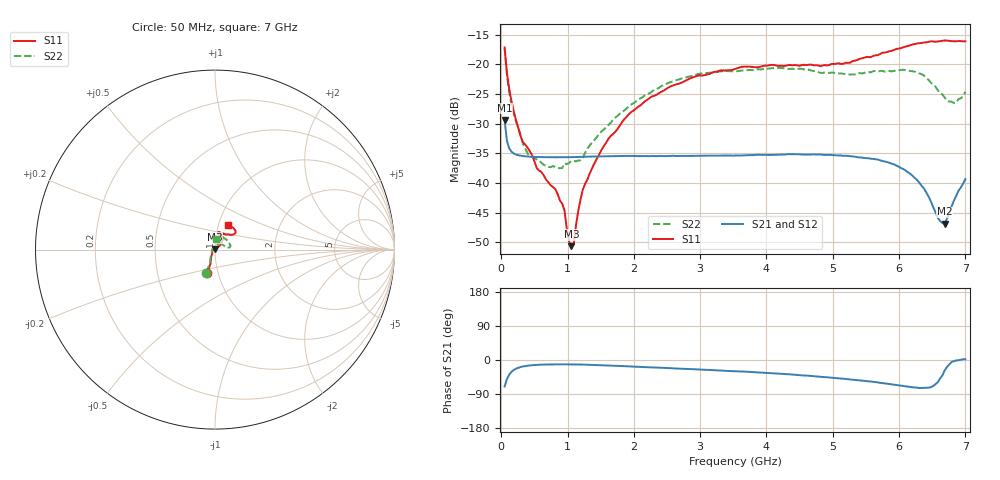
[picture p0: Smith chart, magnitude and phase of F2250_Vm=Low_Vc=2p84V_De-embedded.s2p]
! Integrated Device Technology
! Corporate Headquarters
! 6024 Silver Creek Valley Road
! San Jose, CA 95138  USA
! Phone:  1-408-284-8200
! Toll Free:  1-800-223-1366
! Webpage:  http://www.idt.com/
! Timing and RF Division
! 515 Groton Road, Suite 102
! Westford, MA 01886-6024
! Device:  F2250
! Description: Voltage Variable RF Attenuator
! Frequency:  50.0 -  6000.00 MHz
! Package:  3x3 mm Thin QFN Plastic Package: 16 pin
! Ports:  2 RF, 3 DC
!  Pin  1  = GND
!  Pin  2  = NC
!  Pin  3  = RF1  = Port 1
!  Pin  4  = NC
!  Pin  5  = GND
!  Pin  6  = GND
!  Pin  7  = GND
!  Pin  8  = GND
!  Pin  9  = NC
!  Pin 10  = RF2  = Port 2
!  Pin 11  = NC
!  Pin 12  = GND
!  Pin 13  = GND
!  Pin 14  = VCNTRL
!  Pin 15  = VDD
!  Pin 16  = VMODE
! Vcntrl:  2.840 Volts
! Vmode:  +0.000 Volts
! Vdd:  +3.30  Volts
! Current:  1.175 mA
! Data:  The device was measured on a the F2250 evaluation board which has
!  individual transmission lines to the RF pins.  Data was collected
!  using a calibrated network analyzer.  The evaluation board was
!  de-embedded using a TRL calibration technique.
!  The reference plane is the edge of the package pin.
! Misc:  SN 10
!  Action Tracker AT0258
! Date Measured:  2014-11-26
! Date:  2015-10-15  MJV
! Note:
!  Integrated Device Technology supplies this data as a sample of measured
!  data at the package pin for this product.  Your particular data for this
!  product may vary.
!  Data was taken at 25 degrees C.
!  Integrated Device Technology reserves the right to change this data at anytime.
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# GHz S dB R 50
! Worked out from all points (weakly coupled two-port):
!   201 points, 50 MHz to 7 GHz, reference 50 ohm
!   highest |S21| = -29.41 dB at 50 MHz (marker M1); lowest = -46.9 dB at 6.687 GHz (marker M2)
!   lowest |S11| = -50.7 dB at 1.058 GHz (marker M3), VSWR 1.01, Z = 49.8 + j0.244 ohm
!   |S11| at or under -10 dB: start of sweep to end of sweep
!   |S22| runs from -37.5 to -17.3 dB; largest |S21 - S12| = 6.1e-05
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0.05  -17.18 -108.6  -29.41 -69.8  -29.41 -69.8  -17.28 -111.0
0.08475  -21.45 -107.5  -32.92 -50.4  -32.92 -50.3  -21.74 -110.2
0.15425  -26.24 -116.6  -34.76 -31.2  -34.76 -31.1  -26.82 -122.4
0.29325  -32.21 -127.8  -35.43 -18.5  -35.43 -18.5  -32.10 -137.4
0.3975  -34.09 -141.8  -35.57 -15.0  -35.56 -15.0  -35.05 -160.4
0.91875  -43.52 158.0  -35.69 -11.5  -35.68 -11.5  -37.52 133.5
0.9535  -44.65 169.8  -35.69 -11.5  -35.68 -11.5  -36.66 131.0
1.023  -49.92 143.4  -35.68 -11.6  -35.67 -11.6  -36.63 116.0
1.05775  -50.67 123.3  -35.67 -11.6  -35.67 -11.6  -36.28 110.7
1.0925  -50.42 89.7  -35.65 -11.7  -35.66 -11.7  -36.31 106.2
1.162  -44.67 57.1  -35.64 -11.9  -35.64 -11.9  -36.22 95.5
1.2315  -41.06 44.2  -35.61 -12.1  -35.61 -12.1  -35.78 85.8
1.6485  -32.10 42.0  -35.52 -14.6  -35.52 -14.6  -29.88 64.5
1.96125  -28.04 42.2  -35.46 -17.2  -35.46 -17.2  -26.81 56.8
2.37825  -24.87 47.3  -35.48 -20.3  -35.48 -20.3  -23.99 56.8
3.525  -20.79 72.4  -35.40 -29.5  -35.40 -29.6  -21.19 74.7
4.7065  -20.17 72.3  -35.20 -42.6  -35.20 -42.6  -21.15 72.2
5.85325  -17.81 40.4  -36.63 -63.4  -36.64 -63.5  -21.14 23.0
6.27025  -16.51 40.0  -39.49 -72.8  -39.51 -72.8  -21.37 9.7
6.68725  -15.99 48.7  -46.89 -27.8  -46.88 -27.5  -25.63 28.6
6.861  -16.13 55.1  -42.21 -1.2  -42.17 -1.3  -26.45 57.9
7  -16.13 63.2  -39.36 2.0  -39.33 1.8  -24.63 83.1
